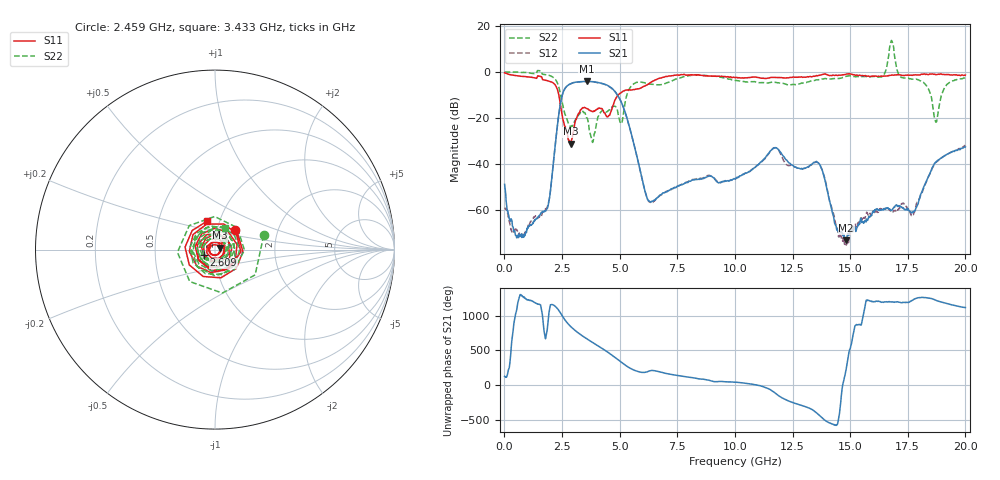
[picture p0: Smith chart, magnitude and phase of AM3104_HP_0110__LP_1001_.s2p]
!Created with skrf (http://scikit-rf.org).
# Hz S RI R 50.0
!freq ReS11 ImS11 ReS21 ImS21 ReS12 ImS12 ReS22 ImS22
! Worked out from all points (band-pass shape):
!   1601 points, 10 MHz to 20 GHz, reference 50 ohm
!   highest |S21| = -4.13 dB at 3.571 GHz (marker M1); lowest = -73.2 dB at 14.83 GHz (marker M2)
!   |S21| within 3 dB of the highest: 2.636 GHz to 4.662 GHz (2.026 GHz wide, 55.5 % of centre)
!   lowest |S11| = -31.2 dB at 2.871 GHz (marker M3), VSWR 1.06, Z = 52.6 + j1.15 ohm
!   |S11| at or under -10 dB: 2.361 GHz to 4.942 GHz (2.582 GHz wide, 70.7 % of centre)
!   |S22| runs from -30.7 to 13.7 dB; largest |S21 - S12| = 0.048
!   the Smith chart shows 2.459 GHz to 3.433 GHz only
!   S11 on the Smith chart (normalised r, x): 2.459 GHz: 1.22, +0.27; 2.609 GHz: 0.88, -0.05; 3.433 GHz: 0.87, +0.29
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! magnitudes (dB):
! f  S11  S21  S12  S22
! 10 MHz  -0.4  -48.9  -59.0  0.0
! 572.2 MHz  -1.7  -71.4  -69.7  -0.1
! 1.809 GHz  -3.7  -60.3  -59.4  -1.2
! 2.459 GHz  -16.1  -12.3  -12.4  -11.0
! 2.609 GHz  -23.4  -7.6  -7.6  -17.7
! 2.871 GHz  -31.2  -5.2  -5.2  -23.9
! 3.346 GHz  -16.1  -4.2  -4.3  -17.0
! 3.433 GHz  -15.6  -4.2  -4.2  -17.6
! 3.571 GHz  -15.9  -4.1  -4.2  -19.9
! 3.821 GHz  -17.2  -4.2  -4.3  -30.6
! 4.92 GHz  -10.2  -10.3  -10.3  -17.5
! 6.182 GHz  -5.7  -54.7  -54.6  -5.1
! 6.682 GHz  -3.0  -54.4  -54.2  -5.6
! 10.01 GHz  -2.5  -46.6  -46.7  -3.7
! 11.72 GHz  -2.4  -33.1  -33.1  -4.5
! 13.34 GHz  -2.1  -40.1  -40.2  -4.0
! 14.83 GHz  -1.0  -73.2  -75.7  -1.9
! 16.38 GHz  -1.8  -59.9  -59.5  -2.1
! 16.68 GHz  -1.6  -59.5  -59.8  7.3
! 17.73 GHz  -1.4  -60.8  -62.1  -3.2
! 18.71 GHz  -1.2  -39.2  -39.4  -21.7
! 20 GHz  -1.4  -32.6  -32.0  -2.6
